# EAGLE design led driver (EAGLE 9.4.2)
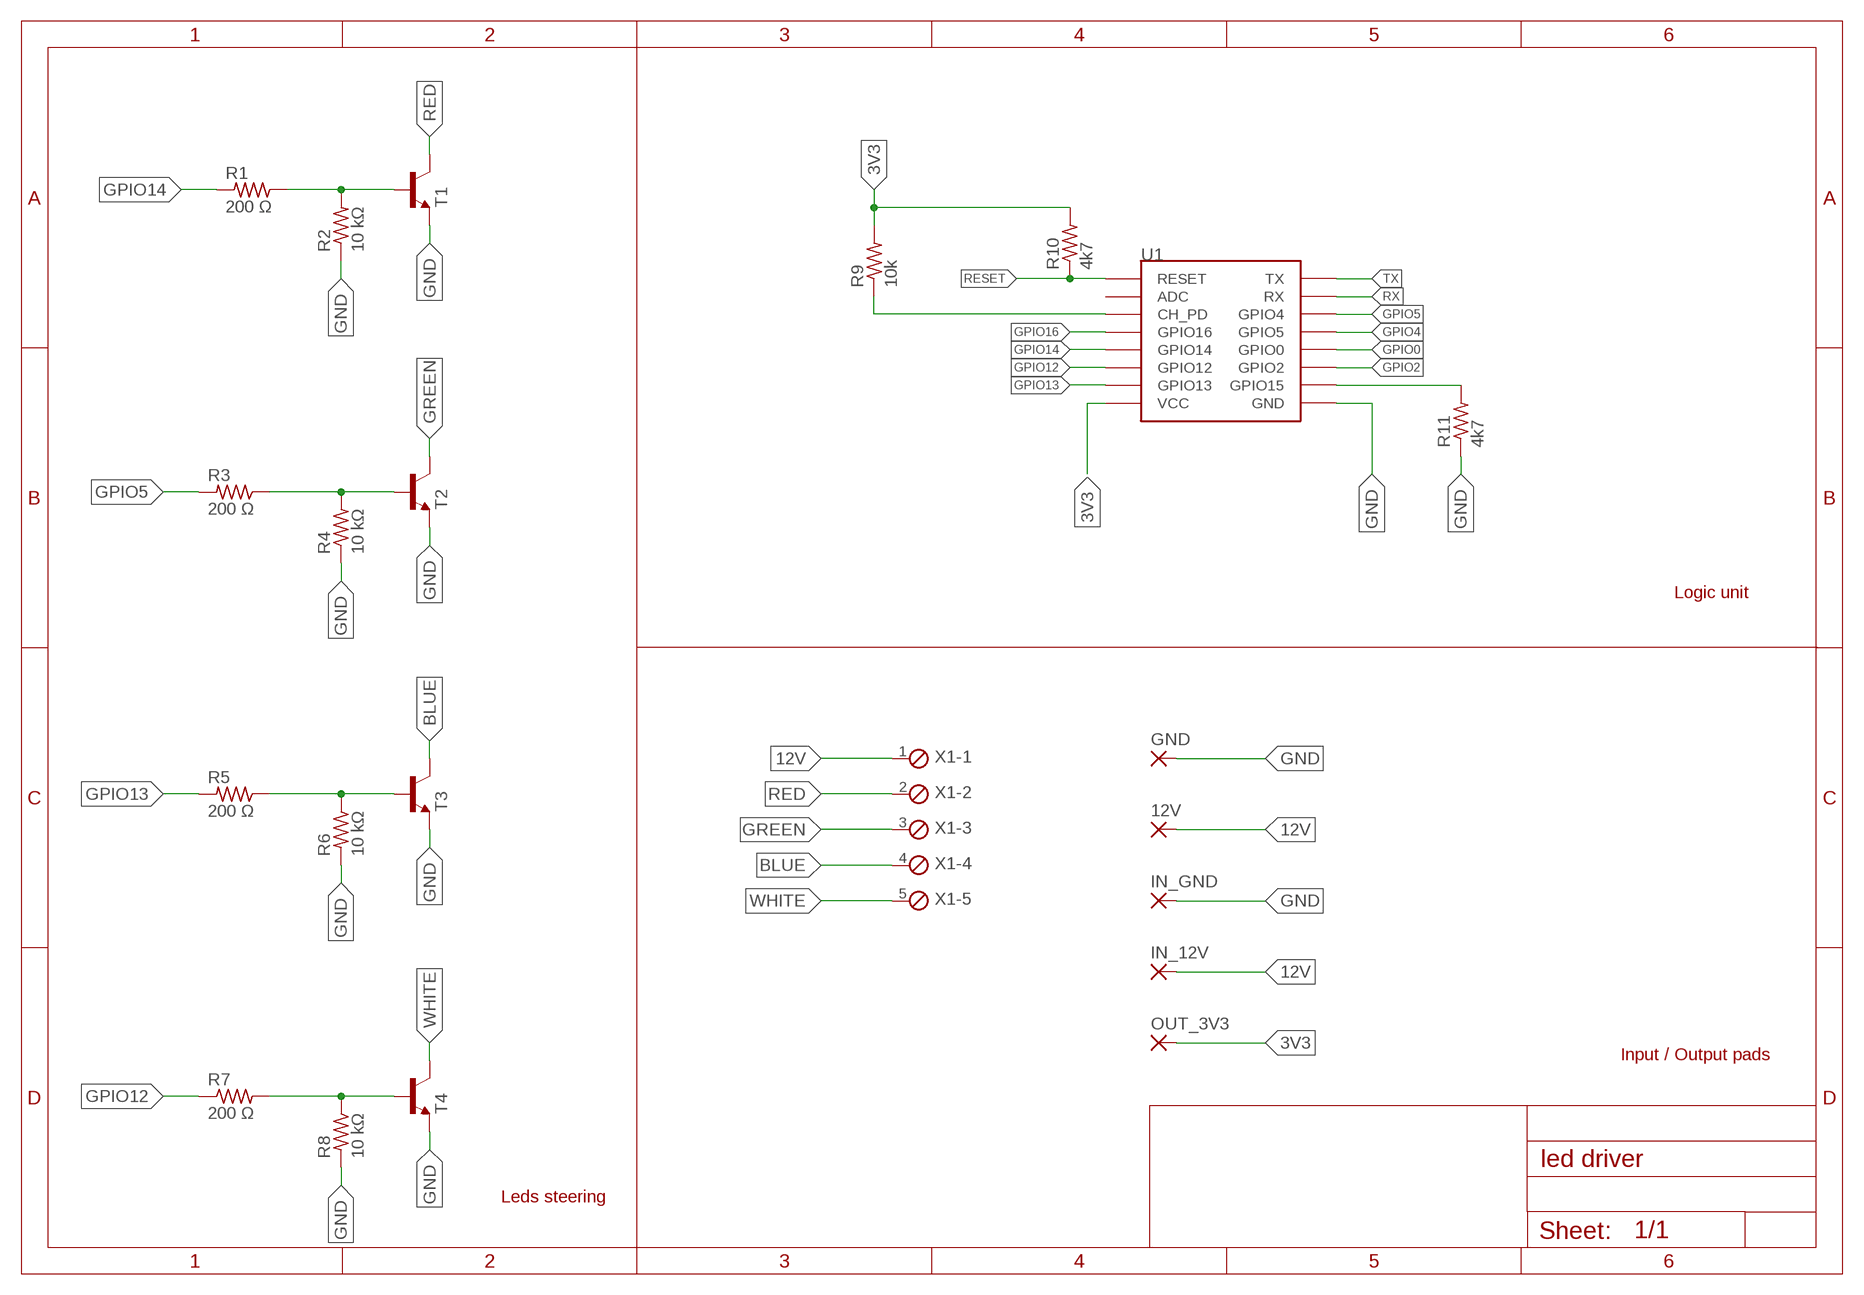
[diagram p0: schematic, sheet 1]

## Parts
12V  WIREPADSMD1,27-254  [SMD1,27-2,54]
GND  WIREPADSMD1,27-254  [SMD1,27-2,54]
IN_12V  WIREPADSMD1,27-254  [SMD1,27-2,54]
IN_GND  WIREPADSMD1,27-254  [SMD1,27-2,54]
OUT_3V3  WIREPADSMD1,27-254  [SMD1,27-2,54]
R1  200 Ω  R-US_R0805  [R0805]
R2  10 kΩ  R-US_R0805  [R0805]
R3  200 Ω  R-US_R0805  [R0805]
R4  10 kΩ  R-US_R0805  [R0805]
R5  200 Ω  R-US_R0805  [R0805]
R6  10 kΩ  R-US_R0805  [R0805]
R7  200 Ω  R-US_R0805  [R0805]
R8  10 kΩ  R-US_R0805  [R0805]
R9  10k  R-US_R0805  [R0805]
R10  4k7  R-US_R0805  [R0805]
R11  4k7  R-US_R0805  [R0805]
T1  BC847B  [SOT23]
T2  BC847B  [SOT23]
T3  BC847B  [SOT23]
T4  BC847B  [SOT23]
U1  ESP12SMD  [ESP12-SMD]
X1  MPT5  [5POL254]

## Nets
3V3 [3V3]: OUT_3V3.1(P) R9.2 R10.2 U1.VCC
12V [12V]: 12V.1(P) IN_12V.1(P) X1.1
BLUE [LED]: T3.3(C) X1.4
GND [GND]: GND.1(P) IN_GND.1(P) R2.1 R4.1 R6.2 R8.2 R11.1 T1.2(E) T2.2(E) T3.2(E) T4.2(E) U1.GND
GPIO0: U1.GPIO0
GPIO2: U1.GPIO2
GPIO4: U1.GPIO5
GPIO5: R3.2 U1.GPIO4
GPIO12: R7.1 U1.GPIO12
GPIO13: R5.2 U1.GPIO13
GPIO14: R1.2 U1.GPIO14
GPIO16: U1.GPIO16
GREEN [LED]: T2.3(C) X1.3
N$1: R1.1 R2.2 T1.1(B)
N$2: R5.1 R6.1 T3.1(B)
N$3: R9.1 U1.CH_PD
N$4: R7.2 R8.1 T4.1(B)
N$5: R3.1 R4.2 T2.1(B)
N$9: R11.2 U1.GPIO15
RED [LED]: T1.3(C) X1.2
RESET: R10.1 U1.RESET
RX: U1.RXD0(RX)
TX: U1.TXD0(TX)
WHITE [LED]: T4.3(C) X1.5
Unconnected: U1.ADC

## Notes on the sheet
- Logic unit
- Input / Output pads
- Leds steering

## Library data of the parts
12V GND IN_12V IN_GND OUT_3V3 = wirepad:WIREPAD: Wire PAD connect wire on PCB
R1-R11 = rcl:R-US_: RESISTOR, American symbol; SPICEPREFIX: R
T1-T4 = NXP_60_26022015:BC847: 45 V, 100 mA NPN general-purpose transistors NPN general-purpose transistor AAL Eindhoven MK
U1 = esp8266modules:ESP12: ESP8266 Wifi module 12
X1 = con-phoenix-254:MPT5: PHOENIX CONNECTOR; OC_FARNELL: unknown; OC_NEWARK: unknown

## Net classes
0 default: width 0.508 mm, drill 0.356 mm, clearance 0.508 mm
1 GND: width 0.508 mm, drill 0.356 mm, clearance 0.508 mm
2 3V3: width 0.508 mm, drill 0.356 mm, clearance 0.508 mm
3 12V: width 1.524 mm, drill 1.372 mm, clearance 0.508 mm
4 LED: width 2.032 mm, drill 1.88 mm, clearance 0.508 mm

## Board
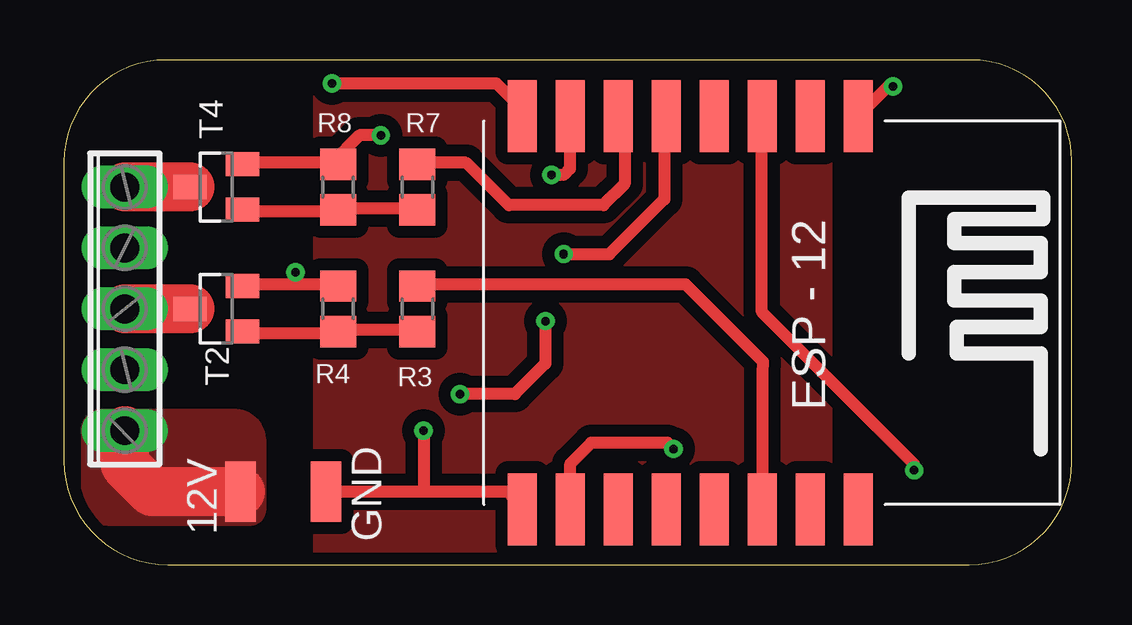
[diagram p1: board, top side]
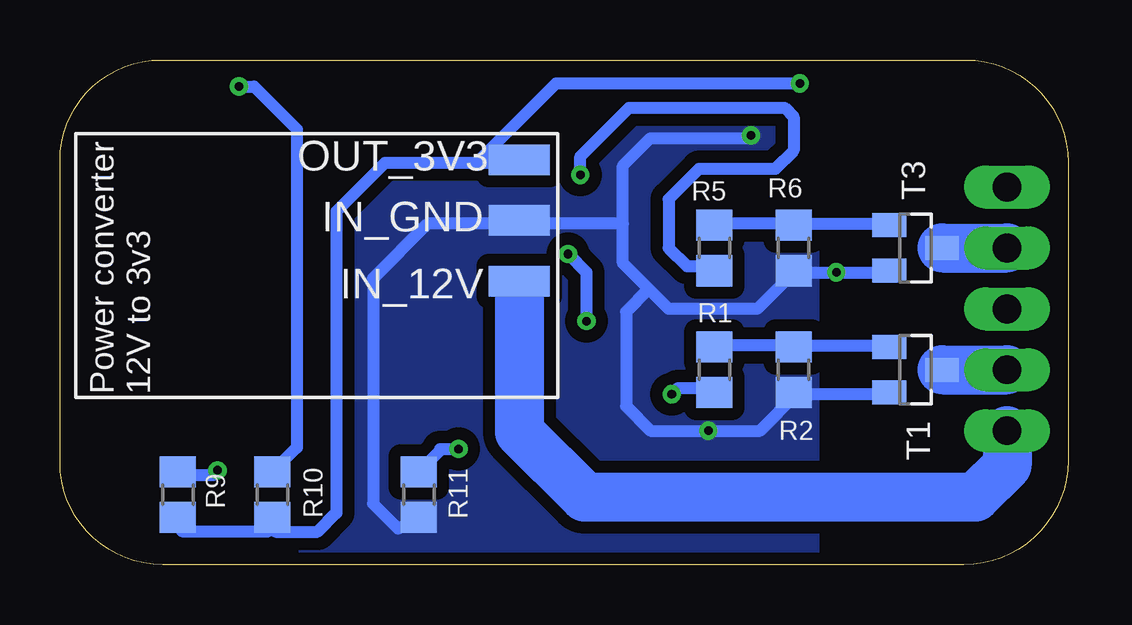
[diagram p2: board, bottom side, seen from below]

Size 42 x 21.05 mm. Coordinates in mm from the lower left corner, seen from the top.
Outline: 4.34,0 37.73,0 arc90 42,4.27 42,16.84 arc90 37.79,21.05 4.27,21.05 arc90 0,16.78 0,4.34 arc90 4.34,0
Copper layers (1*16): Top 0.035mm / dielectric 1.5mm / Bottom 0.035mm
Design rules "default *": minimum track width 6mil, minimum drill 0.35mm, track to track 6mil, track to pad 6mil, pad to pad 6mil, via to via 6mil, smd to smd 6mil, copper to edge 20mil, drill to drill 6mil, minimum pad ring 10mil, minimum via ring 8mil, stop-mask expansion 4mil, vias tented up to drill 0mil, thermal gap 10mil

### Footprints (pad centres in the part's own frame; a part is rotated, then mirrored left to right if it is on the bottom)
SMD1,27-2,54 = smd 1.27 x 2.54: 1 0,0
R0805 = smd 1.3 x 1.5: 1 -0.95,0; 2 0.95,0
SOT23 = smd 1 x 1.4: 1 -0.95,-1.1; 2 0.95,-1.1; 3 0,1.1
ESP12-SMD = smd 3 x 1.2: ADC -8.3,3.8; CH_PD -8.3,1.8; GND 8.1,-8.2; GPIO0 8.1,-2.2; GPIO2 8.1,-4.2; GPIO4 8.1,1.8; GPIO5 8.1,-0.2; GPIO12 -8.3,-4.2; GPIO13 -8.3,-6.2; GPIO14 -8.3,-2.2; GPIO15 8.1,-6.2; GPIO16 -8.3,-0.2; RESET -8.3,5.8; RXD0 8.1,3.8; TXD0 8.1,5.8; VCC -8.3,-8.2
5POL254 = drill 1.2 long: 1 -5.08,0; 2 -2.54,0; 3 0,0; 4 2.54,0; 5 5.08,0

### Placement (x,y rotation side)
12V  7.37,3.05 0 top
GND  10.92,3.05 180 top
IN_12V  22.86,11.81 270 bottom
IN_GND  22.86,14.35 270 bottom
OUT_3V3  22.86,16.89 270 bottom
R1  14.73,8.13 270 bottom
R2  11.43,8.13 90 bottom
R3  14.73,10.67 90 top
R4  11.43,10.67 270 top
R5  14.73,13.21 270 bottom
R6  11.43,13.21 270 bottom
R7  14.73,15.75 270 top
R8  11.43,15.75 90 top
R9  37.08,2.92 270 bottom
R10  33.15,2.92 270 bottom
R11  27.05,2.92 90 bottom
T1  6.35,8.13 270 bottom
T2  6.35,10.67 90 top
T3  6.35,13.21 270 bottom
T4  6.35,15.75 90 top
U1  27.3,10.41 270 top
X1  2.54,10.67 90 top

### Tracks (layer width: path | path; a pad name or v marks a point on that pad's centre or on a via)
3V3  (via drill 0.36)
  Top 0.508: v11.18,20.07 18.03,20.07 18.88,19.23 U1.VCC
  Bottom 0.508: R9.2 36.92,1.4 33.31,1.4 R10.2 33.02,1.37 31.27,1.37 30.48,2.16 30.48,14.73 28.45,16.76 24.64,16.76 | 24.64,16.76 22.86,16.76 OUT_3V3.1 | 24.64,16.76 21.34,20.07 v11.18,20.07
12V
  Top 2.032: 12V.1 3.68,3.05 2.54,4.19 X1.1
  Bottom 1.016: IN_12V.1 22.86,11.43
  Bottom 2.032: X1.1 2.54,4.13 3.85,2.82 20.14,2.82 22.86,5.54 22.86,11.43
  pour Top (no thermals): 8.38,5.18 8.38,2.29 arc-90 7.75,1.65 1.84,1.65 arc-90 0.76,2.73 0.76,5.61 arc-90 1.63,6.48 7.08,6.48 arc-90
BLUE
  Bottom 2.032: T3.3 X1.4
GND  (via drill 0.36)
  Top 0.508: 14.99,3.05 18.51,3.05 U1.GND | 14.99,3.05 GND.1 | 11.18,16.76 11.43,16.76 R8.2 | 11.18,16.76 7.62,16.76 T4.2 | 9.65,11.68 11.43,11.68 R4.1 | 9.65,11.68 7.62,11.68 T2.2 | v9.65,12.19 9.65,11.68 | v13.21,17.91 12.32,17.91 11.18,16.76 | v14.99,5.59 14.99,3.05
  Bottom 0.508: 11.3,7.11 11.43,7.11 R2.1 | 11.3,7.11 7.62,7.11 T1.2 | 11.43,12.19 v9.65,12.19 7.62,12.19 T3.2 | 11.3,7.11 12.83,5.59 v14.99,5.59 17.4,5.59 18.41,6.6 18.41,10.54 17.46,11.49 | 11.43,12.19 12.95,10.67 16.64,10.67 17.46,11.49 | 11.43,12.19 R6.2 | v13.21,17.91 13.34,17.78 17.4,17.78 18.54,16.64 18.54,14.22 | 17.46,11.49 18.54,12.57 18.54,14.22 | 22.86,14.22 26.67,14.22 28.96,11.94 28.96,2.54 27.91,1.5 R11.1 | 18.54,14.22 22.86,14.22 | 22.86,14.22 IN_GND.1
  pour Bottom (no thermals): 10.41,21.08 10.41,0 32,0 32,21.08
GPIO5
  Top 0.508: R3.2 14.99,11.68 25.91,11.68 29.13,8.46 29.11,7.98 U1.GPIO4
GPIO12
  Top 0.508: R7.1 14.8,16.76 16.76,16.76 18.54,14.99 22.48,14.99 23.37,15.88 23.37,18.33 U1.GPIO12
GPIO13  (via drill 0.36)
  Top 0.508: v20.32,16.26 20.83,16.26 21.08,16.51 21.08,18.69 U1.GPIO13
  Bottom 0.508: v20.32,16.26 20.32,17.02 18.29,19.05 11.81,19.05 11.43,18.67 11.43,17.27 12.19,16.51 15.37,16.51 16.64,15.24 16.64,13.21 15.88,12.45 14.73,12.45 R5.2
GPIO14  (via drill 0.36)
  Top 0.508: v20.07,10.16 20.07,8.38 18.8,7.11 v16.51,7.11 | v20.83,12.95 22.73,12.95 25.02,15.24 25.02,18.51 25.15,18.54 U1.GPIO14
  Bottom 0.508: v16.51,7.11 16.26,7.37 14.73,7.37 R1.2 | v20.07,10.16 20.07,12.19 v20.83,12.95
GREEN
  Top 2.032: T2.3 X1.3
N$1
  Bottom 0.508: 11.43,9.14 7.62,9.14 T1.1 | 11.43,9.14 14.73,9.14 R1.1 | 11.43,9.14 R2.2
N$2
  Bottom 0.508: 11.43,14.22 7.62,14.22 T3.1 | 11.43,14.22 14.73,14.22 R5.1 | 11.43,14.22 R6.1
N$3  (via drill 0.36)
  Top 0.508: v35.43,3.94 35.43,4.19 29.08,10.54 29.08,18.69 U1.CH_PD
  Bottom 0.508: R9.1 36.96,3.74 35.63,3.74 v35.43,3.94
N$4
  Top 0.508: T4.1 7.62,14.73 11.43,14.73 R8.1 11.43,14.86 14.73,14.86 R7.2
N$5
  Top 0.508: T2.1 7.62,9.65 11.43,9.65 R4.2 11.43,9.78 14.73,9.78 R3.1
N$6
  pour Top: 10.41,21.08 10.41,0 31.99,0 31.99,21.08
N$9  (via drill 0.36)
  Top 0.508: v25.4,4.83 25.15,5.08 21.97,5.08 21.11,4.21 U1.GPIO15
  Bottom 0.508: v25.4,4.83 26.16,4.83 26.16,4.76 R11.2
RED
  Bottom 2.032: T1.3 X1.2
RESET  (via drill 0.36)
  Top 0.508: v34.54,19.94 34.33,19.94 U1.RESET
  Bottom 0.508: v34.54,19.94 33.91,19.94 32.13,18.16 32.13,4.89 R10.1
WHITE
  Top 2.032: T4.3 X1.5

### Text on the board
bNames: Power converter / 12V to 3v3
